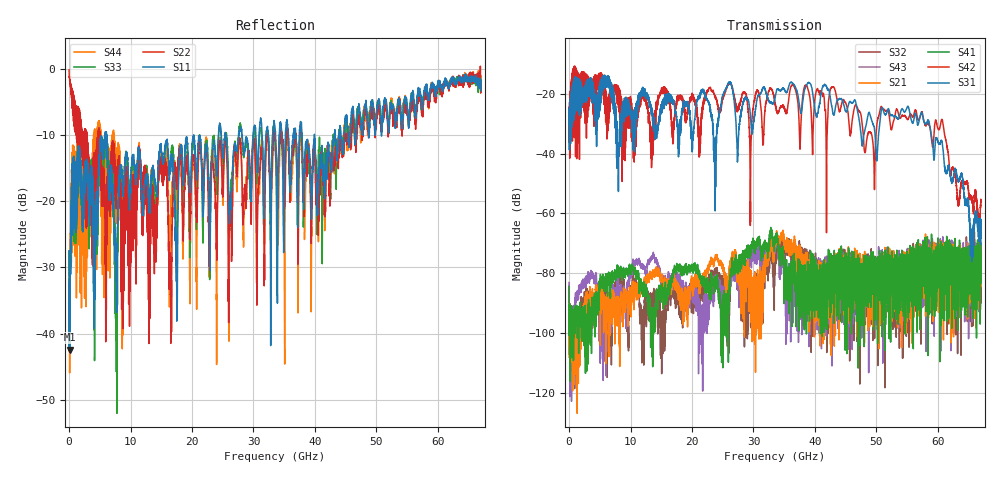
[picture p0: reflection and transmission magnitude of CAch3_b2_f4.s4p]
!Agilent Technologies,N5247A,US51170199,A.09.90.13
!Agilent N5247A: A.09.90.13
!Date: Thursday, October 18, 2018 11:38:33
!Correction: S11(Full 4 Port(1,2,3,4))
!S12(Full 4 Port(1,2,3,4))
!S13(Full 4 Port(1,2,3,4))
!S14(Full 4 Port(1,2,3,4))
!S21(Full 4 Port(1,2,3,4))
!S22(Full 4 Port(1,2,3,4))
!S23(Full 4 Port(1,2,3,4))
!S24(Full 4 Port(1,2,3,4))
!S31(Full 4 Port(1,2,3,4))
!S32(Full 4 Port(1,2,3,4))
!S33(Full 4 Port(1,2,3,4))
!S34(Full 4 Port(1,2,3,4))
!S41(Full 4 Port(1,2,3,4))
!S42(Full 4 Port(1,2,3,4))
!S43(Full 4 Port(1,2,3,4))
!S44(Full 4 Port(1,2,3,4))
!S4P File: Measurements: <S11,S12,S13,S14>,
!<S21,S22,S23,S24>,
!<S31,S32,S33,S34>,
!<S41,S42,S43,S44>:
# Hz S  dB  R 50
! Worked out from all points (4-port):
!   6701 points, 10 MHz to 67 GHz, reference 50 ohm
!   strongest paths, dB at 10 MHz, 16.76 GHz, 33.51 GHz, 50.25 GHz, 67 GHz:
!     S31: -30.3, -22.2, -21.3, -36.4, -68.2
!     S42: -28.7, -31.4, -23.0, -28.3, -56.4
!     S41: -84.6, -81.9, -68.0, -82.4, -76.4
!     S21: -90.4, -80.9, -71.1, -77.2, -73.9
!     S43: -83.1, -82.4, -72.2, -75.0, -74.2
!     S32: -84.1, -85.4, -74.9, -87.8, -76.4
!   lowest |S11| = -42.4 dB at 110 MHz (marker M1), VSWR 1.02, Z = 50.6 + j0.455 ohm
!   |S11| at or under -10 dB: start of sweep to 5.857 GHz; 6.12 GHz to 20.29 GHz (14.17 GHz wide, 107 % of centre); 20.29 GHz to 24.32 GHz (4.031 GHz wide, 18.1 % of centre)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
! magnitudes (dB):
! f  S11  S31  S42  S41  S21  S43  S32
! 10 MHz  -27.5  -30.3  -28.7  -84.6  -90.4  -83.1  -84.1
! 110 MHz  -42.4  -34.0  -41.6  -107.7  -97.5  -97.0  -98.0
! 16.47 GHz  -14.8  -21.1  -25.5  -83.3  -83.3  -82.5  -86.1
! 23.75 GHz  -12.3  -40.3  -21.1  -83.3  -74.8  -81.0  -79.5
! 26.07 GHz  -21.5  -16.0  -16.6  -90.8  -80.4  -85.5  -92.1
! 55.07 GHz  -6.2  -24.3  -28.5  -75.2  -85.7  -88.6  -79.7
! 67 GHz  -3.4  -68.2  -56.4  -76.4  -73.9  -74.2  -76.4
